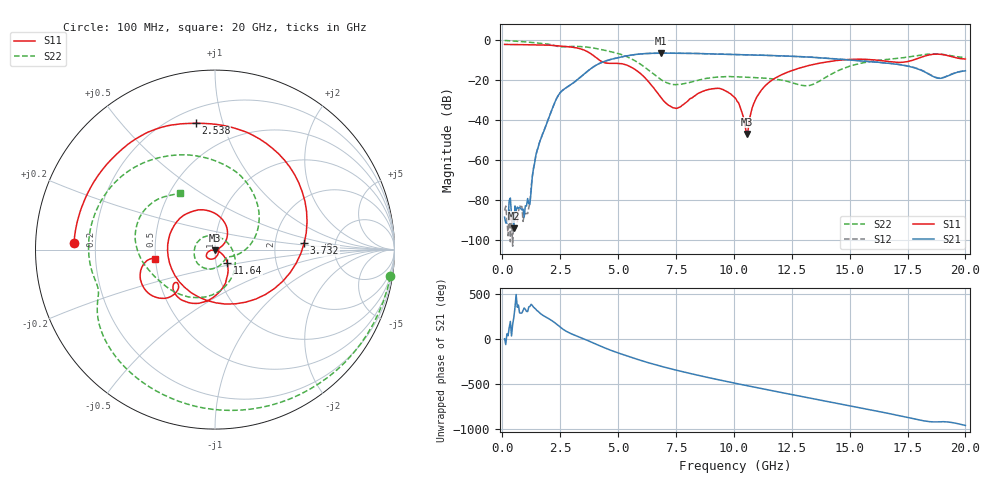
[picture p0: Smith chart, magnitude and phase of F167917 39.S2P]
!  2-Port S-parameters saved by WinCal
! VAR MeasName=S-Parameters (CALIBRATED_DATA) read from VNA (N5242A)
! VAR MeasDate=2016-11-22 9:01:41
! VAR NAME=F167917 39
! VAR FILENAME=F167917 39.S2P
! VAR DATE=2016-11-22 9:01:41
! VAR PHYS_PORTS=1,2
# Hz S DB R 50
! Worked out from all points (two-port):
!   401 points, 100 MHz to 20 GHz, reference 50 ohm
!   highest |S21| = -6.44 dB at 6.866 GHz (marker M1); lowest = -94.0 dB at 498 MHz (marker M2)
!   |S21| within 3 dB of the highest: 4.733 GHz to 14.51 GHz (9.773 GHz wide, 102 % of centre)
!   lowest |S11| = -46.8 dB at 10.55 GHz (marker M3), VSWR 1.01, Z = 49.8 - j0.401 ohm
!   |S11| at or under -10 dB: 4.204 GHz to 14.52 GHz (10.31 GHz wide, 110 % of centre); 16.24 GHz to 17.72 GHz (1.48 GHz wide, 8.72 % of centre)
!   |S22| runs from -22.7 to -0.1 dB; largest |S21 - S12| = 0.0042
!   S11 on the Smith chart (normalised r, x): 100 MHz: 0.12, +0.02; 2.538 GHz: 0.29, +0.82; 3.732 GHz: 2.96, +0.29; 11.64 GHz: 1.13, -0.17; 20 GHz: 0.49, -0.06
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1e8  -2.09 177.3  -88.42 5.6  -85.06 164.6  -0.10 -8.7
4.98e8  -2.14 166.7  -93.96 -117.9  -87.04 171.5  -0.36 -40.7
1.14475e9  -2.25 149.1  -81.63 -0.4  -83.62 -0.2  -0.96 -87.5
1.54275e9  -2.34 137.2  -53.80 -48.8  -53.50 -48.9  -1.38 -112.7
2.53775e9  -2.95 98.8  -25.70 127.1  -25.71 126.9  -3.27 -162.0
3.43325e9  -4.49 38.5  -17.88 12.9  -17.89 13.0  -3.19 158.8
3.73175e9  -6.05 4.2  -15.00 -19.0  -15.00 -18.8  -3.52 144.0
4.1795e9  -9.81 -69.1  -11.69 -69.6  -11.63 -69.6  -4.42 121.9
4.72675e9  -11.57 -171.5  -9.46 -126.9  -9.41 -127.1  -5.82 95.1
5.62225e9  -13.79 91.2  -7.31 153.8  -7.32 153.5  -9.54 43.6
6.7665e9  -27.27 26.9  -6.44 65.3  -6.46 65.3  -18.98 -17.8
6.866e9  -28.79 24.6  -6.44 58.5  -6.46 58.4  -19.76 -21.3
8.06e9  -29.71 -61.8  -6.53 -17.7  -6.53 -17.7  -21.25 -66.0
9.254e9  -24.01 -131.0  -6.90 -86.3  -6.88 -86.4  -18.42 -122.9
1.005e10  -28.76 -163.0  -7.09 -129.3  -7.10 -129.3  -18.25 -151.3
1.05475e10  -46.82 -118.1  -7.25 -155.4  -7.26 -155.5  -18.48 -165.2
1.099525e10  -28.29 -30.0  -7.41 -178.6  -7.40 -178.6  -18.74 -176.9
1.1642e10  -19.98 -47.0  -7.62 148.0  -7.61 148.2  -19.24 163.3
1.338325e10  -12.22 -86.2  -8.51 59.2  -8.45 59.5  -22.20 33.5
1.67165e10  -10.66 -140.5  -11.51 -107.6  -11.53 -107.8  -9.45 -140.3
1.885575e10  -6.96 -156.7  -18.99 160.7  -18.86 160.3  -6.86 153.0
2e10  -9.36 -170.9  -15.23 120.4  -15.15 119.9  -8.62 121.4
